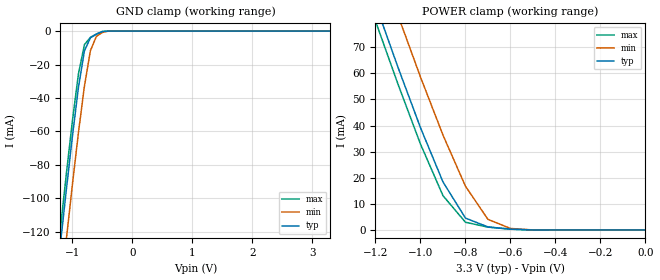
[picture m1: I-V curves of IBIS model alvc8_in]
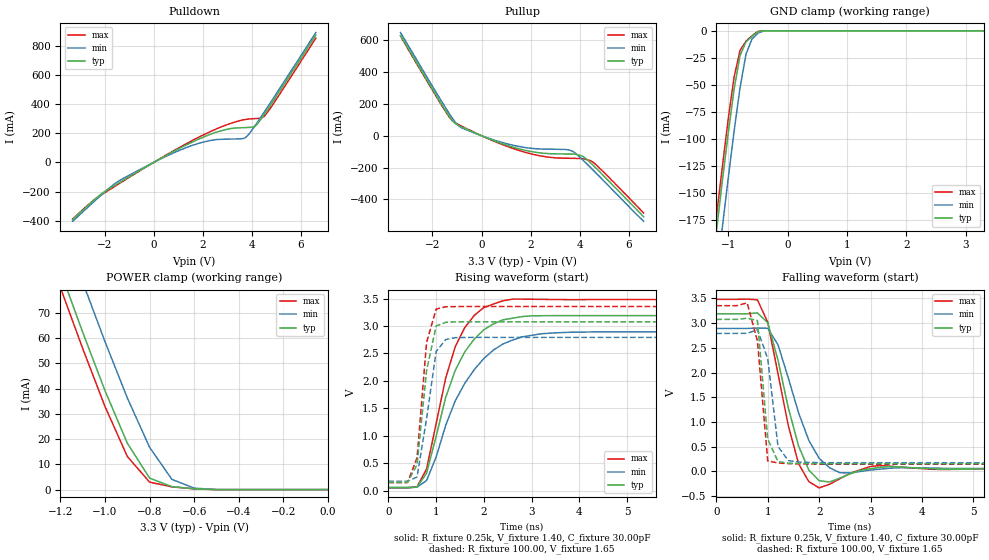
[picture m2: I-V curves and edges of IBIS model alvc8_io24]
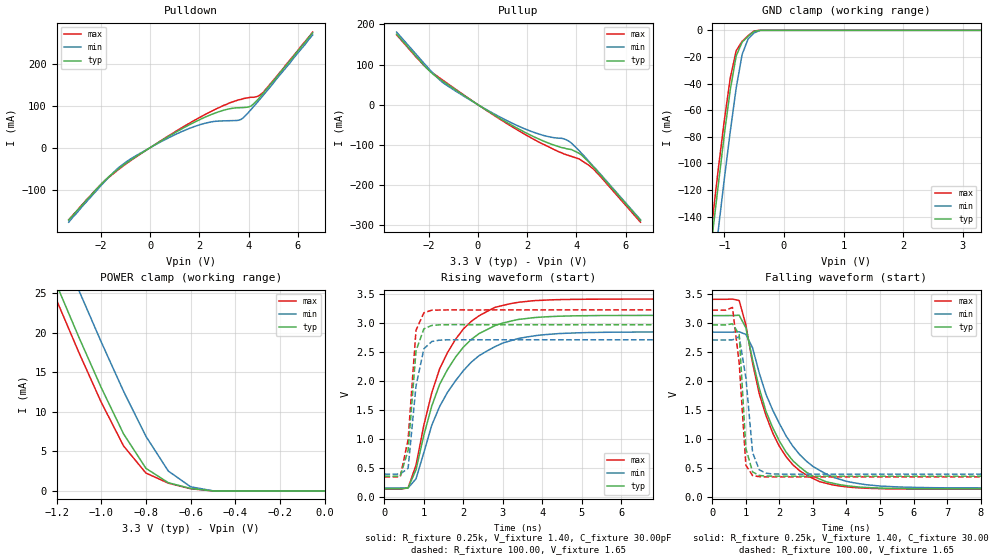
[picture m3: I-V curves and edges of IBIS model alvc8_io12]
| IBIS file 162245a.ibs created by s2ibis2 version 1.1
| North Carolina State University Electronics Research Laboratory  1995
[IBIS ver]   2.1
[File name]   162245a.ibs
[File Rev]   1.0
[Date]   03/01/99 rtk rtk
[Source]   Integrated Device Technology, Inc.
[Notes]   1.Temperatures: typ=25C, min=100C, max=0C 2.RRmp rates based
   on 50 ohm load.
[Disclaimer] Integrated Device Technology, Inc. ("IDT") hereby grants the
   user of this IBIS model a non-exclusive, nontransferable
   license to use this IBIS model under the following terms. The
   user is granted this license only to use the IBIS model and is
   not granted rights to sell, copy (except as needed to run the
   IBIS model), rent, lease or sub-license the IBIS model in
   whole or in part, or in modified form to anyone. The User may
   modify the IBIS model to suit its specific applications, but
   rights to derivative works and such modifications shall belong
   to IDT. This IBIS model is provided on an AS IS" basis and IDT
   makes absolutely no warranty with respect to the information
   contained herein. IDT DISCLAIMS AND CUSTOMER WAIVES ALL
   WARRANTIES, EXPRESS AND IMPLIED, INCLUDING WARRANTIES OF
   MERCHANTABILITY AND FITNESS FOR A PARTICULAR PURPOSE. THE
   ENTIRE RISK AS TO QUALITY AND PERFORMANCE IS WITH THE USER
   ACCORDINGLY, IN NO EVENT SHALL IDT BE LIABLE FOR ANY DIRECT OR
   INDIRECT DAMAGES, WHETHER IN CONTRACT OR TORT, INCLUDING ANY
   LOST PROFITS OR OTHER INCIDENTAL, CONSEQUENTIAL, EXEMPLARY, OR
   PUNITIVE DAMAGES ARISING OUT OF THE USE OR APPLICATION OF THE
   IBIS model. Further, IDT reserves the right to make changes
   without notice to any product herein to improve reliability,
   function, or design. IDT does not convey any license under
   patent rights or any other intellectual property rights,
   including those of third parties. IDT is not obligated to
   provide maintenance or support for the licensed IBIS model.
[Copyright]   Copyright 1997, Integrated Device Technology, Inc. all rights
   reserved
|   Component ALVC162245
[Component]   ALVC162245
[Manufacturer]   Integrated Device Technology
[Package]
|PA48
| variable   typ   min   max
R_pkg   6.50m   5.00m   10.00m
L_pkg   3.20nH   2.50nH   4.40nH
C_pkg   0.27pF   0.01pF   0.98pF
| PV48   typ   min   max
|R_pkg   6.5m   5.00m   10.00m
|L_pkg   4.75nH   3.82nH   6.72nH
|C_pkg   0.24pF   0.01pF   1.55pF
[Pin]  signal_name   model_name   R_pin   L_pin   C_pin
1   1DIR   alvc8_in
2   1B1   alvc8_io24
3   1B2   alvc8_io24
4   GND   GND
5   1B3   alvc8_io24
6   1B4   alvc8_io24
7   VCC   POWER
8   1B5   alvc8_io24
9   1B6   alvc8_io24
10   GND   GND
11   1B7   alvc8_io24
12   1B8   alvc8_io24
13   2B1   alvc8_io24
14   2B2   alvc8_io24
15   GND   GND
16   2B3   alvc8_io24
17   2B4   alvc8_io24
18   VCC   POWER
19   2B5   alvc8_io24
20   2B6   alvc8_io24
21   GND   GND
22   2B7   alvc8_io24
23   2B8   alvc8_io24
24   2DIR   alvc8_in
25   2OEB   alvc8_in
26   2A8   alvc8_io12
27   2A7   alvc8_io12
28   GND   GND
29   2A6   alvc8_io12
30   2A5   alvc8_io12
31   VCC   POWER
32   2A4   alvc8_io12
33   2A3   alvc8_io12
34   GND   GND
35   2A2   alvc8_io12
36   2A1   alvc8_io12
37   1A8   alvc8_io12
38   1A7   alvc8_io12
39   GND   GND
40   1A6   alvc8_io12
41   1A5   alvc8_io12
42   VCC   POWER
43   1A4   alvc8_io12
44   1A3   alvc8_io12
45   GND   GND
46   1A2   alvc8_io12
47   1A1   alvc8_io12
48   1OEB   alvc8_in
| Models and submodels in the file (3): alvc8_in (Input), alvc8_io24 (I/O), alvc8_io12 (I/O)
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| in   in   dummy_model
| oe   oe   dummy_model
|   Model alvc8_in
[Model]   alvc8_in
Model_type   Input
Vinl =  0.800V
Vinh =  2.000V
C_comp   3.00pF   NA   NA
[Temperature Range]   25.00   100.00   0.000
[Voltage Range]   3.30V   3.00V   3.60V
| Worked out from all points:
|   GND clamp passes 1 mA (typ) near -0.54 V on its own axis
|   POWER clamp passes 1 mA (typ) near -0.68 V on its own axis
[GND_clamp]
| voltage   I(typ)   I(min)   I(max)
-3.3V     -860mA     -887mA     -851mA
-1.3V     -161mA     -190mA     -151mA
-1.2V     -127mA     -157mA     -118mA
-1.1V     -94.41mA   -124mA     -84.85mA
-1V       -62.78mA   -91.54mA   -53.52mA
-900mV    -33.71mA   -60.78mA   -25.6mA
-800mV    -11.74mA   -32.83mA   -8.09mA
-700mV    -4.033mA   -11.65mA   -3.7mA
-600mV    -1.899mA   -3.108mA   -1.699mA
-500mV    -308uA     -810uA     -172uA
-400mV    -3.848nA   -9.872uA   -399pA
3.3V      39.6pA     19.33nA    26.4pA
[POWER_clamp]
| voltage   I(typ)   I(min)   I(max)
-3.3V     630mA      648mA      624mA
-1.2V     86.56mA    106mA      80.02mA
-1.1V     62.33mA    82.22mA    55.88mA
-1V       39.2mA     58.61mA    32.91mA
-900mV    18.4mA     36.35mA    13.15mA
-800mV    4.556mA    16.76mA    2.954mA
-700mV    1.164mA    4.056mA    1.087mA
-600mV    320uA      578uA      299uA
-500mV    40.08nA    12.23uA    3.465nA
0V        39.6pA     59.11pA    43.2pA
|   Model alvc8_io24
[Model]   alvc8_io24
Model_type   I/O
Polarity   Non-Inverting
Enable   Active-High
Vinl =  0.000V
Vinh =  2.000V
Vmeas =  1.500V
C_comp   3.00pF   NA   NA
[Temperature Range]   25.00   100.00   0.000
[Voltage Range]   3.30V   3.00V   3.60V
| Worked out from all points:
|   slope of the pulldown table from 0 to 0.495 V, typ, clamps not added: 10.5 ohm
|   slope of the pullup table from 0 to 0.495 V, typ, clamps not added: 16.1 ohm
|   GND clamp passes 1 mA (typ) near -0.50 V on its own axis
|   POWER clamp passes 1 mA (typ) near -0.68 V on its own axis
|   rising waveform, R_fixture 0.25k, V_fixture 1.40, C_fixture 30.00pF: 20-80 % time 720ps typ, 913ps min, 616ps max; typ from 0.056 V to 3.19 V
|   rising waveform, R_fixture 100.00, V_fixture 1.65: 20-80 % time 244ps typ, 272ps min, 186ps max; typ from 0.155 V to 3.08 V
|   falling waveform, R_fixture 0.25k, V_fixture 1.40, C_fixture 30.00pF: 20-80 % time 438ps typ, 529ps min, 406ps max; typ from 3.19 V to 0.056 V
|   falling waveform, R_fixture 100.00, V_fixture 1.65: 20-80 % time 146ps typ, 176ps min, 172ps max; typ from 3.08 V to 0.155 V
[Pulldown]
| voltage   I(typ)   I(min)   I(max)
-3.3V     -392mA     -404mA     -388mA
-2.3V     -240mA     -249mA     -241mA
-1.5V     -149mA     -136mA     -156mA
300mV     28.7mA     25.4mA     30.2mA
1.4V      126mA      107mA      135mA
2.3V      193mA      151mA      211mA
3.1V      232mA      161mA      266mA
3.6V      239mA      163mA      291mA
3.8V      240mA      180mA      297mA
4.1V      246mA      246mA      301mA
4.5V      329mA      345mA      316mA
6.6V      875mA      892mA      853mA
[Pullup]
| voltage   I(typ)   I(min)   I(max)
-3.3V     630mA      649mA      628mA
-1.4V     142mA      160mA      137mA
-1.1V     80.6mA     90.7mA     83.6mA
-900mV    63mA       57.7mA     67.6mA
400mV     -25.1mA    -21.5mA    -27.4mA
1.6V      -85mA      -69.5mA    -95.9mA
2.6V      -111mA     -84mA      -132mA
3.4V      -115mA     -86.1mA    -141mA
3.7V      -115mA     -97.1mA    -142mA
4.1V      -128mA     -149mA     -144mA
4.5V      -179mA     -210mA     -162mA
6.6V      -510mA     -538mA     -486mA
[GND_clamp]
| voltage   I(typ)   I(min)   I(max)
-3.3V     -1.238A    -1.278A    -1.225A
-1.3V     -235mA     -278mA     -221mA
-1.2V     -187mA     -230mA     -173mA
-1.1V     -140mA     -183mA     -127mA
-1V       -95.25mA   -137mA     -82.01mA
-900mV    -53.91mA   -92.86mA   -42.75mA
-800mV    -22.78mA   -52.64mA   -18.06mA
-700mV    -10.26mA   -21.65mA   -9.608mA
-600mV    -5.099mA   -7.641mA   -4.562mA
-500mV    -851uA     -2.177mA   -482uA
-400mV    -8.815nA   -25.71uA   -702pA
3.3V      106pA      19.43nA    92.4pA
[POWER_clamp]
| voltage   I(typ)   I(min)   I(max)
-3.3V     630mA      648mA      624mA
-1.2V     86.56mA    106mA      80.02mA
-1.1V     62.33mA    82.22mA    55.88mA
-1V       39.2mA     58.61mA    32.91mA
-900mV    18.4mA     36.35mA    13.15mA
-800mV    4.556mA    16.76mA    2.954mA
-700mV    1.164mA    4.056mA    1.087mA
-600mV    320uA      578uA      299uA
-500mV    40.16nA    12.23uA    3.547nA
0V        106pA      150pA      115pA
[Ramp]
| variable   typ   min   max
dV/dt_r   1.48/0.31n   1.29/0.30n   1.66/0.22n
dV/dt_f   1.63/0.28n   1.45/0.31n   1.80/0.19n
R_load = 50.00
[Rising Waveform]
R_fixture = 0.25k
V_fixture = 1.40
C_fixture = 30.00pF
R_dut = 7.00m
L_dut = 3.30nH
C_dut = 0.29pF
| time   V(typ)   V(min)   V(max)
0s        55.61mV    62.15mV    53.22mV
600ps     66.97mV    63.74mV    71.16mV
800ps     321mV      187mV      397mV
1ns       990mV      613mV      1.221V
1.2ns     1.699V     1.191V     2.052V
1.4ns     2.193V     1.637V     2.622V
1.8ns     2.764V     2.207V     3.194V
2.4ns     3.112V     2.673V     3.459V
3.8ns     3.189V     2.886V     3.48V
19.8ns    3.189V     2.893V     3.481V
[Rising Waveform]
R_fixture = 100.00
V_fixture = 1.65
R_dut = 7.00m
L_dut = 3.30nH
C_dut = 0.29pF
| time   V(typ)   V(min)   V(max)
0s        155mV      173mV      149mV
400ps     155mV      173mV      149mV
600ps     473mV      251mV      599mV
800ps     2.188V     1.312V     2.7V
1ns       3V         2.535V     3.306V
1.2ns     3.067V     2.753V     3.351V
1.4ns     3.075V     2.787V     3.353V
1.8ns     3.077V     2.793V     3.355V
19.8ns    3.076V     2.792V     3.354V
[Falling Waveform]
R_fixture = 0.25k
V_fixture = 1.40
C_fixture = 30.00pF
R_dut = 7.00m
L_dut = 3.30nH
C_dut = 0.29pF
| time   V(typ)   V(min)   V(max)
0s        3.189V     2.893V     3.481V
800ps     3.206V     2.901V     3.472V
1ns       3.01V      2.896V     3.019V
1.2ns     2.252V     2.563V     1.978V
1.4ns     1.288V     1.891V     927mV
1.6ns     514mV      1.185V     156mV
2ns       -189mV     264mV      -333mV
2.4ns     -138mV     -26.28mV   -151mV
3.2ns     83.76mV    47.29mV    118mV
19.8ns    55.61mV    62.15mV    53.22mV
[Falling Waveform]
R_fixture = 100.00
V_fixture = 1.65
R_dut = 7.00m
L_dut = 3.30nH
C_dut = 0.29pF
| time   V(typ)   V(min)   V(max)
0s        3.076V     2.792V     3.354V
400ps     3.076V     2.793V     3.354V
600ps     3.1V       2.794V     3.41V
800ps     3.053V     2.868V     2.639V
1ns       655mV      2.284V     212mV
1.2ns     198mV      503mV      171mV
1.4ns     168mV      219mV      157mV
1.6ns     161mV      191mV      153mV
2ns       156mV      177mV      149mV
19.8ns    155mV      173mV      149mV
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|   Model alvc8_io12
[Model]   alvc8_io12
Model_type   I/O
Polarity   Non-Inverting
Enable   Active-High
Vinl =  0.000V
Vinh =  2.000V
Vmeas =  1.500V
C_comp   3.00pF   NA   NA
[Temperature Range]   25.00   100.00   0.000
[Voltage Range]   3.30V   3.00V   3.60V
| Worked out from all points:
|   slope of the pulldown table from 0 to 0.495 V, typ, clamps not added: 27.6 ohm
|   slope of the pullup table from 0 to 0.495 V, typ, clamps not added: 25.8 ohm
|   GND clamp passes 1 mA (typ) near -0.51 V on its own axis
|   POWER clamp passes 1 mA (typ) near -0.69 V on its own axis
|   rising waveform, R_fixture 0.25k, V_fixture 1.40, C_fixture 30.00pF: 20-80 % time 1.05ns typ, 1.21ns min, 974ps max; typ from 0.138 V to 3.12 V
|   rising waveform, R_fixture 100.00, V_fixture 1.65: 20-80 % time 182ps typ, 253ps min, 198ps max; typ from 0.356 V to 2.96 V
|   falling waveform, R_fixture 0.25k, V_fixture 1.40, C_fixture 30.00pF: 20-80 % time 1.11ns typ, 1.35ns min, 1.03ns max; typ from 3.12 V to 0.138 V
|   falling waveform, R_fixture 100.00, V_fixture 1.65: 20-80 % time 159ps typ, 240ps min, 228ps max; typ from 2.96 V to 0.356 V
[Pulldown]
| voltage   I(typ)   I(min)   I(max)
-3.3V     -172mA     -177mA     -171mA
-1.8V     -75.8mA    -78mA      -76.8mA
-1.3V     -51.3mA    -48.6mA    -52.8mA
-600mV    -22.3mA    -20mA      -23.2mA
800mV     28.5mA     25mA       30mA
1.9V      63.5mA     52.4mA     68.3mA
3V        89.4mA     63.9mA     101mA
3.7V      95.4mA     67.5mA     115mA
4.1V      99.1mA     90.7mA     120mA
4.4V      116mA      111mA      123mA
4.6V      130mA      125mA      132mA
6.6V      273mA      268mA      275mA
[Pullup]
| voltage   I(typ)   I(min)   I(max)
-3.3V     176mA      181mA      174mA
-1.9V     80.3mA     83.6mA     82mA
-1.5V     61.8mA     58.9mA     64.3mA
-1V       40.8mA     37.7mA     42.5mA
400mV     -15.6mA    -14.2mA    -16.4mA
1.7V      -62.2mA    -54.9mA    -66.6mA
2.9V      -96.6mA    -80.2mA    -106mA
3.5V      -108mA     -85.3mA    -123mA
3.8V      -112mA     -96mA      -129mA
4.2V      -125mA     -121mA     -139mA
4.7V      -156mA     -155mA     -161mA
6.6V      -289mA     -287mA     -293mA
[GND_clamp]
| voltage   I(typ)   I(min)   I(max)
-3.3V     -1.018A    -1.051A    -1.008A
-1.3V     -193mA     -229mA     -182mA
-1.2V     -154mA     -189mA     -143mA
-1.1V     -116mA     -150mA     -104mA
-1V       -78.53mA   -112mA     -67.94mA
-900mV    -44.74mA   -76.24mA   -35.91mA
-800mV    -19.2mA    -43.26mA   -15.27mA
-700mV    -8.824mA   -17.98mA   -8.247mA
-600mV    -4.484mA   -6.51mA    -4.028mA
-500mV    -777uA     -1.948mA   -445uA
-400mV    -8.815nA   -25.33uA   -702pA
3.3V      106pA      19.43nA    92.4pA
[POWER_clamp]
| voltage   I(typ)   I(min)   I(max)
-3.3V     175mA      181mA      173mA
-1.3V     32.91mA    38.88mA    30.95mA
-1.2V     26.11mA    32.08mA    24.16mA
-1.1V     19.45mA    25.38mA    17.52mA
-1V       13.07mA    18.85mA    11.22mA
-900mV    7.211mA    12.6mA     5.686mA
-800mV    2.858mA    6.904mA    2.259mA
-700mV    1.039mA    2.515mA    986uA
-600mV    306uA      524uA      278uA
-500mV    40.16nA    12.11uA    3.547nA
0V        106pA      150pA      115pA
[Ramp]
| variable   typ   min   max
dV/dt_r   1.29/0.24n   1.13/0.30n   1.44/0.25n
dV/dt_f   1.26/0.26n   1.08/0.26n   1.40/0.24n
R_load = 50.00
[Rising Waveform]
R_fixture = 0.25k
V_fixture = 1.40
C_fixture = 30.00pF
R_dut = 7.00m
L_dut = 3.30nH
C_dut = 0.29pF
| time   V(typ)   V(min)   V(max)
0s        138mV      152mV      132mV
600ps     153mV      154mV      155mV
800ps     465mV      310mV      545mV
1.2ns     1.564V     1.234V     1.792V
1.4ns     1.938V     1.557V     2.206V
2ns       2.577V     2.172V     2.889V
2.8ns     2.948V     2.585V     3.262V
3.8ns     3.086V     2.772V     3.378V
5.2ns     3.119V     2.829V     3.403V
19.8ns    3.124V     2.839V     3.405V
[Rising Waveform]
R_fixture = 100.00
V_fixture = 1.65
R_dut = 7.00m
L_dut = 3.30nH
C_dut = 0.29pF
| time   V(typ)   V(min)   V(max)
0s        356mV      391mV      343mV
400ps     356mV      392mV      344mV
600ps     797mV      492mV      988mV
800ps     2.514V     1.907V     2.868V
1ns       2.893V     2.55V      3.17V
1.2ns     2.951V     2.674V     3.213V
1.4ns     2.961V     2.698V     3.216V
2ns       2.964V     2.704V     3.218V
19.8ns    2.963V     2.704V     3.218V
[Falling Waveform]
R_fixture = 0.25k
V_fixture = 1.40
C_fixture = 30.00pF
R_dut = 7.00m
L_dut = 3.30nH
C_dut = 0.29pF
| time   V(typ)   V(min)   V(max)
0s        3.124V     2.839V     3.405V
800ps     3.13V      2.845V     3.384V
1ns       2.913V     2.8V       2.961V
1.2ns     2.358V     2.567V     2.302V
1.4ns     1.868V     2.131V     1.773V
1.8ns     1.192V     1.494V     1.101V
2.4ns     623mV      873mV      553mV
3.2ns     307mV      456mV      262mV
5.6ns     143mV      169mV      136mV
19.8ns    138mV      153mV      132mV
[Falling Waveform]
R_fixture = 100.00
V_fixture = 1.65
R_dut = 7.00m
L_dut = 3.30nH
C_dut = 0.29pF
| time   V(typ)   V(min)   V(max)
0s        2.963V     2.704V     3.218V
400ps     2.963V     2.704V     3.218V
600ps     2.982V     2.705V     3.264V
800ps     2.799V     2.761V     2.305V
1ns       832mV      2.05V      544mV
1.2ns     429mV      762mV      366mV
1.4ns     368mV      465mV      347mV
1.6ns     358mV      407mV      344mV
1.8ns     357mV      394mV      343mV
19.8ns    356mV      391mV      343mV
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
